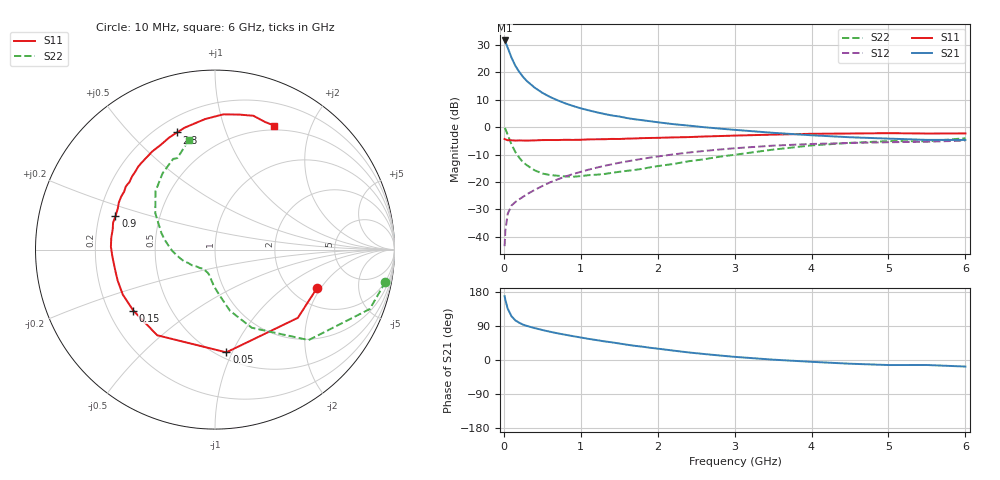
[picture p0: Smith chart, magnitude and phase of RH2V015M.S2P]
! SIEMENS Small Signal Semiconductors
! BFR106
! Si NPN RF Bipolar Junction Transistor in SOT23
! VCE = 2 V  IC = 15 mA
! Common Emitter S-Parameters:  August  1996
# GHz  S  MA  R  50
!  f  S11  S21  S12  S22
! GHz  MAG  ANG  MAG  ANG  MAG  ANG  MAG  ANG
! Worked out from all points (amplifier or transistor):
!   36 points, 10 MHz to 6 GHz, reference 50 ohm
!   highest |S21| = 31.5 dB at 10 MHz (marker M1)
!   |S21| within 3 dB of that: start of sweep to 54.89 MHz
!   unconditionally stable (mu >= 1): 392.8 MHz to 2.467 GHz; 5.051 GHz to end of sweep
!   at 250 MHz: K = 0.84, MSG = 21.8 dB, |S12| = -25.4 dB
!   at 1.4 GHz: K = 1.09, MAG = 7.1 dB, |S12| = -13.6 dB
!   at 6 GHz: K = 1.02, MAG = -0.7 dB, |S12| = -4.9 dB
!   S11 on the Smith chart (normalised r, x): 10 MHz: 2.73, -1.84; 50 MHz: 0.55, -0.95; 150 MHz: 0.30, -0.30; 900 MHz: 0.27, +0.15; 2.8 GHz: 0.28, +0.69; 6 GHz: 0.45, +1.49
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0.01  0.6077 -20.5  37.74 168.4  0.0068 82.5  0.9667 -10.7
0.02  0.598 -39.5  35.89 158.8  0.0132 73.5  0.9239 -21.0
0.05  0.576 -83.7  27.83 135.5  0.0264 58.0  0.7257 -44.0
0.1  0.5758 -124.0  18.32 115.4  0.0374 49.2  0.4812 -64.8
0.15  0.568 -143.3  13.04 104.5  0.0433 47.7  0.3512 -76.2
0.2  0.5716 -154.0  10.13 98.3  0.0485 49.6  0.278 -81.9
0.25  0.5693 -162.3  8.174 93.3  0.0539 51.3  0.2289 -87.7
0.3  0.5676 -167.3  6.872 89.9  0.0599 54.2  0.202 -91.9
0.4  0.5727 -175.7  5.231 84.2  0.0717 57.2  0.1635 -98.4
0.5  0.5802 178.5  4.21 79.2  0.0845 59.6  0.1429 -103.6
0.6  0.5817 173.4  3.54 74.6  0.0986 61.0  0.134 -108.2
0.7  0.5809 168.8  3.064 70.4  0.1118 61.7  0.1302 -113.3
0.9  0.5847 161.5  2.421 62.9  0.1398 61.6  0.1245 -121.5
1.1  0.5964 153.9  2.021 55.8  0.1676 60.5  0.1331 -129.9
1.3  0.6006 147.4  1.74 49.4  0.1961 58.7  0.1395 -137.7
1.6  0.6163 138.6  1.46 40.4  0.2371 55.5  0.1598 -148.9
2.2  0.6491 122.5  1.132 24.9  0.318 47.3  0.2127 -170.6
2.8  0.6862 108.0  0.941 12.0  0.3899 37.9  0.2885 168.4
3.5  0.7292 94.4  0.786 0.9  0.4593 26.8  0.3892 148.7
4.5  0.7641 79.9  0.653 -9.8  0.5143 11.4  0.5158 124.5
5.5  0.7636 68.4  0.585 -13.2  0.5417 1.8  0.5513 112.3
6  0.7662 64.4  0.584 -17.3  0.5677 -5.3  0.6265 103.6
